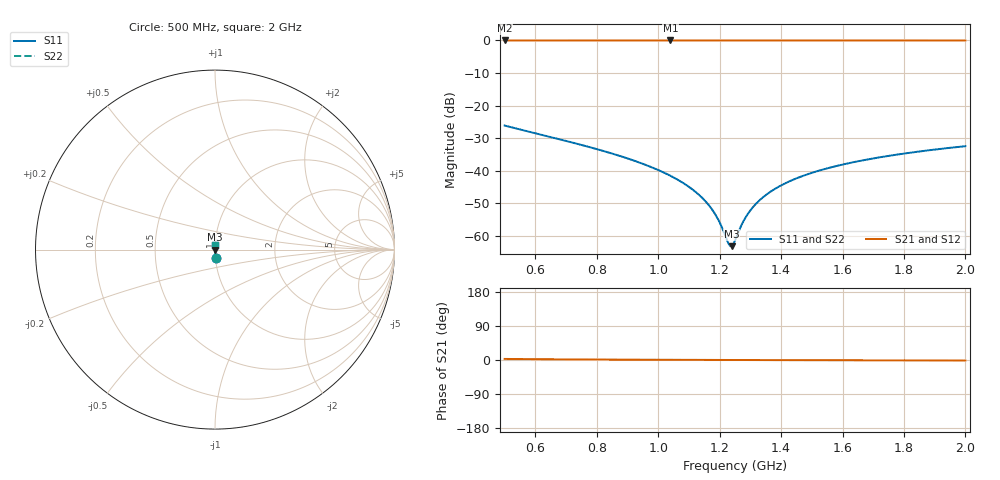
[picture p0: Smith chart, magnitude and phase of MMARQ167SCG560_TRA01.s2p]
! MMARQ167SCG560_TRA01  S-PARAMETER MODEL  ( General Type )
! Model Generated by TAIYO YUDEN Corporation (http://www.ty-top.com)
! Version 1.0
! TAIYO YUDEN Control No. 150305
! Copyright(c) 2015 TAIYO YUDEN CO.,LTD. All Rights Reserved.
! Product Description (link to TY-COMPAS)
! https://ds.yuden.co.jp/TYCOMPAS/or/detail?pn=MMARQ167SCG560JTRA01&u=M
! Products Name : Multilayer Ceramic Capacitors
! Characteristics :
!  Capacitance : 56 pF , Rated Voltage : 250V , TCC : CG / C0G
!  Case Size : 1.6 x 0.8 / 0.063 x 0.031 [mm/inch] , Thickness : 0.7 / 0.028 [mm/inch]
!  (Conditions: Temperature = 25 degC , DC Bias Current/Voltage = 0A / 0V)
! External Node Assignments :
!  1  o---| |---o  2
! GND o---------o GND
! Frequency Range : 500MHz  -  2GHz  [ 401 STEP ]
# MHz S RI R 50
! Freq[MHz].  S11 Real  S11 Imag  S21 Real  S21 Imag  S12 Real  S12 Imag  S22 Real  S22 Imag
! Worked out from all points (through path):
!   401 points, 500 MHz to 2 GHz, reference 50 ohm
!   highest |S21| = -0.01 dB at 1.04 GHz (marker M1); lowest = 0.0 dB at 500 MHz (marker M2)
!   lowest |S11| = -63.1 dB at 1.239 GHz (marker M3), VSWR 1.00, Z = 50.1 + j0.00525 ohm
!   |S11| at or under -10 dB: start of sweep to end of sweep
!   |S22| runs from -63.1 to -26.1 dB; largest |S21 - S12| = 0
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500  0.00296 -0.0494  0.997 0.0494  0.997 0.0494  0.00296 -0.0494
751.25  0.00115 -0.0249  0.9989 0.0249  0.9989 0.0249  0.00115 -0.0249
893.75  0.00081 -0.0158  0.9992 0.0158  0.9992 0.0158  0.00081 -0.0158
1002.5  0.000697 -0.0102  0.9993 0.0102  0.9993 0.0102  0.000697 -0.0102
1040  0.000677 -0.00836  0.9993 0.00836  0.9993 0.00836  0.000677 -0.00836
1107.5  0.000663 -0.00532  0.9993 0.00532  0.9993 0.00532  0.000663 -0.00532
1156.25  0.000668 -0.00325  0.9993 0.00325  0.9993 0.00325  0.000668 -0.00325
1186.25  0.000675 -0.00202  0.9993 0.00202  0.9993 0.00202  0.000675 -0.00202
1201.25  0.000681 -0.00142  0.9993 0.00142  0.9993 0.00142  0.000681 -0.00142
1227.5  0.000692 -0.000384  0.9993 0.000384  0.9993 0.000384  0.000692 -0.000384
1238.75  0.000698 5.24e-05  0.9993 -5.24e-05  0.9993 -5.24e-05  0.000698 5.24e-05
1250  0.000704 0.000485  0.9993 -0.000485  0.9993 -0.000485  0.000704 0.000485
1272.5  0.000717 0.00134  0.9993 -0.00134  0.9993 -0.00134  0.000717 0.00134
1287.5  0.000727 0.0019  0.9993 -0.0019  0.9993 -0.0019  0.000727 0.0019
1310  0.000744 0.00273  0.9993 -0.00273  0.9993 -0.00273  0.000744 0.00273
1336.25  0.000765 0.00368  0.9992 -0.00368  0.9992 -0.00368  0.000765 0.00368
1370  0.000795 0.00488  0.9992 -0.00488  0.9992 -0.00488  0.000795 0.00488
1407.5  0.000833 0.00618  0.9992 -0.00618  0.9992 -0.00618  0.000833 0.00618
1501.25  0.000942 0.00931  0.9991 -0.00931  0.9991 -0.00931  0.000942 0.00931
1613.75  0.0011 0.0129  0.9989 -0.0129  0.9989 -0.0129  0.0011 0.0129
1752.5  0.00133 0.017  0.9987 -0.017  0.9987 -0.017  0.00133 0.017
2000  0.00183 0.0238  0.9982 -0.0238  0.9982 -0.0238  0.00183 0.0238
